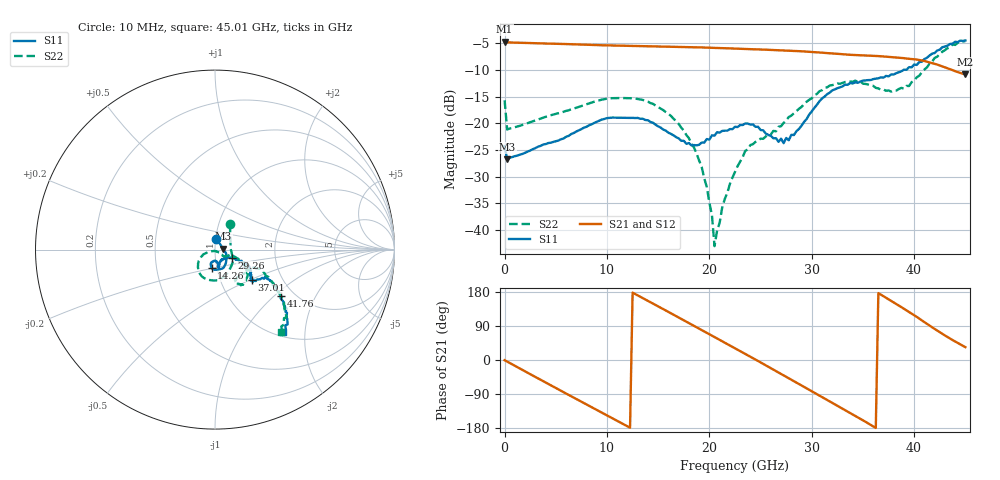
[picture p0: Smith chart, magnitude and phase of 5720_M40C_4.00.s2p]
! Device:  ADRF5720
! Description: 0.5dB LSB GaAs MMIC 6-bit Digital Attenuator
! Frequency:  0.000009 -  40 GHz
! Ports:
!	RF1	= Port 1
!	RF2	= Port 2
! Vdd:  3.3 Volt
! Vss:  -3.3 Volt
! Control:  0/3.3 Volt
! State:  4.00 dB attenuation
! Data:  The device was measured using G-S-G Probes on a matrix board.
!  Data was collected using an calibrated 4 port network analyzer.
!  The reference plane for this measurement is at the launchers.
! Note:  Analog Devices supplies this data as a sample of measured data
!  for this product.  Your particular data for this product may vary.
!  Data was taken at -40 degrees C.
!  Analog Devices reserves the right to change this data at anytime.
# GHZ S DB R 45.0
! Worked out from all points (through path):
!   181 points, 10 MHz to 45.01 GHz, reference 45 ohm
!   highest |S21| = -4.68 dB at 10 MHz (marker M1); lowest = -10.8 dB at 45.01 GHz (marker M2)
!   group delay of S21, straight-line fit = 42 ps
!   lowest |S11| = -26.8 dB at 260 MHz (marker M3), VSWR 1.10, Z = 49.3 + j0.46 ohm
!   |S11| at or under -10 dB: start of sweep to 38.97 GHz
!   |S22| runs from -43.0 to -4.6 dB; largest |S21 - S12| = 0.0022
!   S11 on the Smith chart (normalised r, x): 10 MHz: 1.01, +0.12; 14.26 GHz: 0.94, -0.19; 29.26 GHz: 1.20, -0.11; 37.01 GHz: 1.41, -0.52; 41.76 GHz: 1.70, -1.11; 45.01 GHz: 1.08, -1.54
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0.01  -24.28 82.5  -4.68 -0.6  -4.70 -0.6  -15.69 59.6
0.26  -26.76 5.8  -4.84 -4.1  -4.86 -4.1  -21.18 1.6
4.26  -23.72 -18.6  -5.06 -62.9  -5.08 -63.0  -18.63 -31.6
7.76  -20.82 -46.5  -5.26 -113.8  -5.28 -113.8  -16.60 -62.7
11.26  -18.97 -76.1  -5.47 -164.2  -5.48 -164.3  -15.28 -95.2
14.26  -19.76 -100.4  -5.58 152.4  -5.60 152.4  -16.22 -124.2
15.26  -20.82 -104.8  -5.61 137.8  -5.63 137.8  -17.23 -133.7
18.76  -24.15 -89.4  -5.77 86.4  -5.78 86.3  -25.70 -159.4
19.76  -22.96 -81.5  -5.82 71.7  -5.84 71.5  -31.97 -155.8
20.26  -22.26 -78.6  -5.85 64.2  -5.87 64.1  -37.27 -140.9
20.51  -22.32 -77.9  -5.87 60.5  -5.89 60.4  -43.04 -106.5
21.26  -21.44 -75.3  -5.92 49.4  -5.93 49.3  -35.78 -47.5
22.76  -20.72 -79.5  -6.02 27.1  -6.04 27.1  -28.05 -35.2
24.01  -20.25 -77.7  -6.11 8.6  -6.13 8.5  -24.09 -37.2
27.26  -23.73 -53.9  -6.34 -40.4  -6.36 -40.5  -19.92 -19.6
29.26  -19.74 -26.8  -6.54 -71.0  -6.56 -71.2  -16.41 -23.4
30.26  -17.12 -23.4  -6.66 -86.5  -6.69 -86.6  -14.76 -28.1
34.01  -12.54 -35.2  -7.19 -143.8  -7.22 -143.9  -12.22 -49.1
37.01  -11.44 -39.5  -7.47 168.4  -7.49 168.2  -13.68 -56.5
37.76  -10.85 -37.6  -7.59 156.1  -7.62 155.9  -14.08 -51.8
41.76  -6.96 -35.3  -8.71 86.5  -8.74 86.3  -8.45 -30.4
45.01  -4.48 -50.5  -10.82 33.8  -10.86 33.7  -4.61 -51.4
